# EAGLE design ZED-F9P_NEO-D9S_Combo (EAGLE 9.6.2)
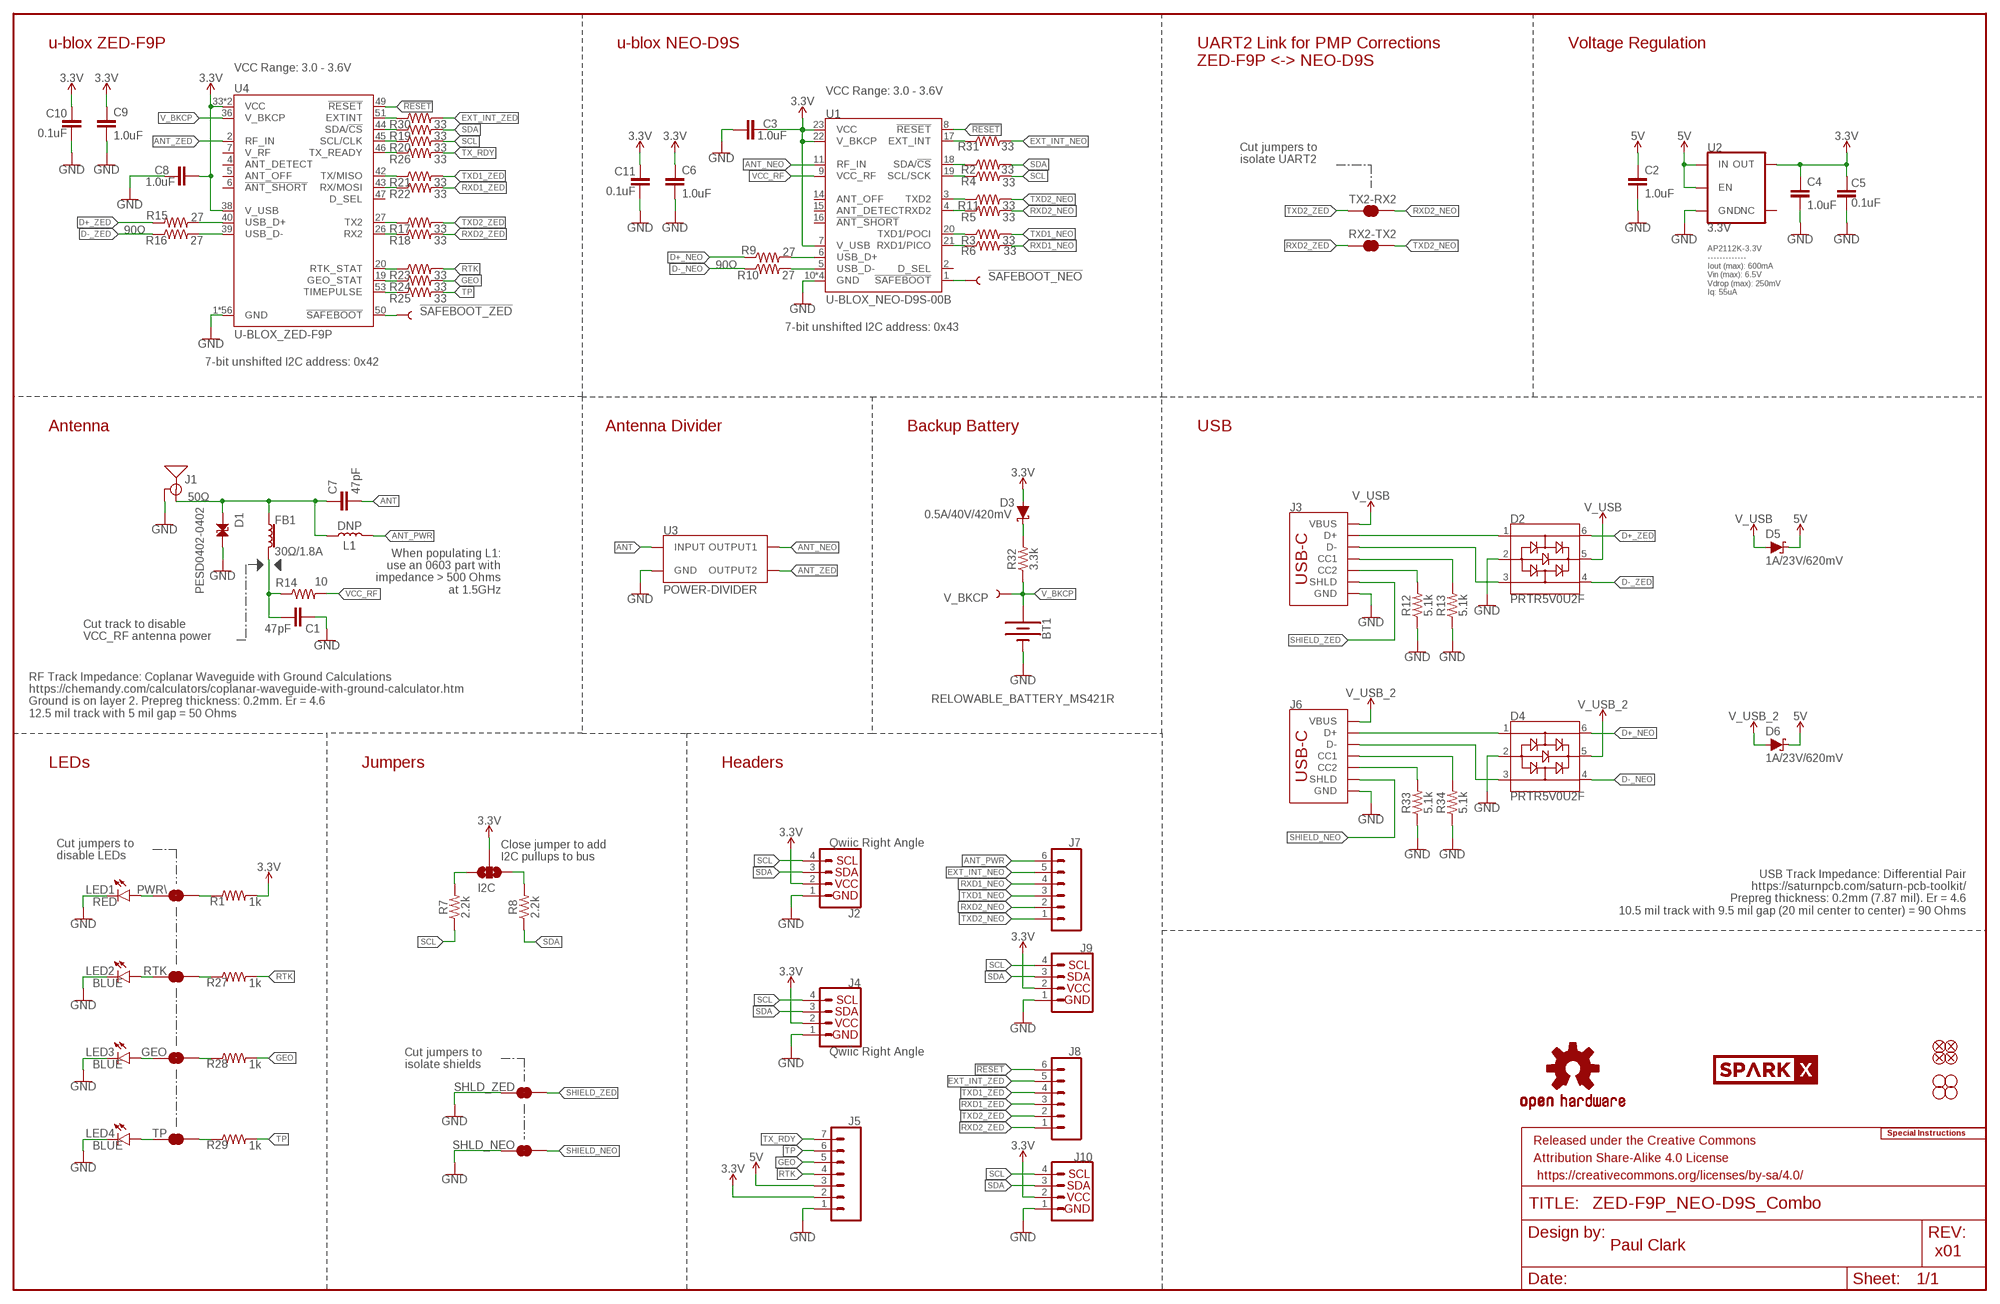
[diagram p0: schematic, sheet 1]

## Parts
!SAFEBOOT_NEO!  TEST-POINTPOGO_PTH  [1X01_NO_SILK]
!SAFEBOOT_ZED!  TEST-POINTPOGO_PTH  [1X01_NO_SILK]
BT1  RELOWABLE_BATTERY_MS421R  [MS421R_IV03E]
C1  47pF  47PF-0603-50V-5%  [0603]
C2  1.0uF  1.0UF-0603-16V-10%  [0603]
C3  1.0uF  1.0UF-0603-16V-10%  [0603]
C4  1.0uF  1.0UF-0603-16V-10%  [0603]
C5  0.1uF  0.1UF-0603-25V-(+80/-20%)  [0603]
C6  1.0uF  1.0UF-0603-16V-10%  [0603]
C7  47pF  47PF-0603-50V-5%  [0603]
C8  1.0uF  1.0UF-0603-16V-10%  [0603]
C9  1.0uF  1.0UF-0603-16V-10%  [0603]
C10  0.1uF  0.1UF-0603-25V-(+80/-20%)  [0603]
C11  0.1uF  0.1UF-0603-25V-(+80/-20%)  [0603]
D1  PESD0402-0402  [0402]
D2  PRTR5V0U2F  [SOT886]
D3  0.5A/40V/420mV  DIODE-SCHOTTKY-PMEG4005EJ  [SOD-323]
D4  PRTR5V0U2F  [SOT886]
D5  1A/23V/620mV  DIODE-SCHOTTKY-BAT20J  [SOD-323]
D6  1A/23V/620mV  DIODE-SCHOTTKY-BAT20J  [SOD-323]
FB1  30Ω/1.8A  FERRITE_BEAD-0603  [0603]
FRAME2  FRAME-LEDGER  [CREATIVE_COMMONS]
GEO  JUMPER-SMT_2_NC_TRACE_SILK  [SMT-JUMPER_2_NC_TRACE_SILK]
I2C  JUMPER-SMT_3_NO_SILK  [SMT-JUMPER_3_NO_SILK]
J1  ANTENNA-SMA-GROUNDEDEDGE_SMA  [SMA-EDGE]
J2  Qwiic Right Angle  I2C_STANDARDQWIIC  [JST04_1MM_RA]
J3  USB Female Type C Connector  USB_C_4-LAYER_PADS  [USB-C-16P_4LAYER-PADS]
J4  Qwiic Right Angle  I2C_STANDARDQWIIC  [JST04_1MM_RA]
J5  CONN_07NO_SILK  [1X07_NO_SILK]
J6  USB Female Type C Connector  USB_C_4-LAYER_PADS  [USB-C-16P_4LAYER-PADS]
J7  CONN_06NO_SILK_FEMALE_PTH  [1X06_NO_SILK]
J8  CONN_06NO_SILK_FEMALE_PTH  [1X06_NO_SILK]
J9  I2C_STANDARD_NO_SILK  [1X04_NO_SILK]
J10  I2C_STANDARD_NO_SILK  [1X04_NO_SILK]
JP21  FIDUCIALUFIDUCIAL  [MICRO-FIDUCIAL]
JP31  STAND-OFF  [STAND-OFF]
JP41  STAND-OFF  [STAND-OFF]
JP61  FIDUCIALUFIDUCIAL  [MICRO-FIDUCIAL]
JP71  FIDUCIALUFIDUCIAL  [MICRO-FIDUCIAL]
JP81  FIDUCIALUFIDUCIAL  [MICRO-FIDUCIAL]
JP91  STAND-OFF  [STAND-OFF]
JP101  STAND-OFF  [STAND-OFF]
L1  DNP  DNP-0603_NO-CREAM  [0603_NO-CREAM]
LED1  RED  LED-RED0603  [LED-0603]
LED2  BLUE  LED-BLUE0603  [LED-0603]
LED3  BLUE  LED-BLUE0603  [LED-0603]
LED4  BLUE  LED-BLUE0603  [LED-0603]
LOGO4  OSHW-LOGOS  [OSHW-LOGO-S]
LOGO5  SPECIAL_INSTRUCTIONS-ORDERING  [ORDERING_INSTRUCTIONS]
PWR\  JUMPER-SMT_2_NC_TRACE_SILK  [SMT-JUMPER_2_NC_TRACE_SILK]
R1  1k  1KOHM-0603-1/10W-1%  [0603]
R2  33  33OHM-0603-1/10W-1%  [0603]
R3  33  33OHM-0603-1/10W-1%  [0603]
R4  33  33OHM-0603-1/10W-1%  [0603]
R5  33  33OHM-0603-1/10W-1%  [0603]
R6  33  33OHM-0603-1/10W-1%  [0603]
R7  2.2k  2.2KOHM-0603-1/10W-1%  [0603]
R8  2.2k  2.2KOHM-0603-1/10W-1%  [0603]
R9  27  27OHM-0603-1/10W-1%  [0603]
R10  27  27OHM-0603-1/10W-1%  [0603]
R11  33  33OHM-0603-1/10W-1%  [0603]
R12  5.1k  5.1KOHM5.1KOHM-0603-1/10W-1%  [0603]
R13  5.1k  5.1KOHM5.1KOHM-0603-1/10W-1%  [0603]
R14  10  10OHM-0603-1/10W-1%  [0603]
R15  27  27OHM-0603-1/10W-1%  [0603]
R16  27  27OHM-0603-1/10W-1%  [0603]
R17  33  33OHM-0603-1/10W-1%  [0603]
R18  33  33OHM-0603-1/10W-1%  [0603]
R19  33  33OHM-0603-1/10W-1%  [0603]
R20  33  33OHM-0603-1/10W-1%  [0603]
R21  33  33OHM-0603-1/10W-1%  [0603]
R22  33  33OHM-0603-1/10W-1%  [0603]
R23  33  33OHM-0603-1/10W-1%  [0603]
R24  33  33OHM-0603-1/10W-1%  [0603]
R25  33  33OHM-0603-1/10W-1%  [0603]
R26  33  33OHM-0603-1/10W-1%  [0603]
R27  1k  1KOHM-0603-1/10W-1%  [0603]
R28  1k  1KOHM-0603-1/10W-1%  [0603]
R29  1k  1KOHM-0603-1/10W-1%  [0603]
R30  33  33OHM-0603-1/10W-1%  [0603]
R31  33  33OHM-0603-1/10W-1%  [0603]
R32  3.3k  3.3KOHM-0603-1/10W-1%  [0603]
R33  5.1k  5.1KOHM5.1KOHM-0603-1/10W-1%  [0603]
R34  5.1k  5.1KOHM5.1KOHM-0603-1/10W-1%  [0603]
RTK  JUMPER-SMT_2_NC_TRACE_SILK  [SMT-JUMPER_2_NC_TRACE_SILK]
RX2-TX2  JUMPER-SMT_2_NC_TRACE_SILK  [SMT-JUMPER_2_NC_TRACE_SILK]
SHLD_NEO  JUMPER-SMT_2_NC_TRACE_SILK  [SMT-JUMPER_2_NC_TRACE_SILK]
SHLD_ZED  JUMPER-SMT_2_NC_TRACE_SILK  [SMT-JUMPER_2_NC_TRACE_SILK]
TP  JUMPER-SMT_2_NC_TRACE_SILK  [SMT-JUMPER_2_NC_TRACE_SILK]
TX2-RX2  JUMPER-SMT_2_NC_TRACE_SILK  [SMT-JUMPER_2_NC_TRACE_SILK]
U1  U-BLOX_NEO-D9S-00B  [NEO-M9N/M8T/M8U/D9S]
U2  3.3V  V_REG_AP2112K-3.3V  [SOT23-5]
U3  POWER-DIVIDER  [PD0922J5050S2HF_ANA]
U4  U-BLOX_ZED-F9P  [ZED-F9P]
U$77  SPARKX-LOGO4  [SPARKX-MEDIUM]
U$78  SPARKX-LOGO4  [SPARKX-MEDIUM]
V_BKCP  TEST-POINT3X5  [PAD.03X.05]

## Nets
3.3V [3.3V]: C3.1 C4.1 C5.2 C6.1 C8.2 C9.1 C10.2 C11.2 D3.A I2C.2 J2.2 J4.2 J5.2 J9.2 J10.2 R1.2 U1.7(V_USB) U1.22(V_BKCP) U1.23(VCC) U2.5(OUT) U4.33(VCC) U4.34(VCC) U4.38(V_USB)
5V: C2.1 D5.C D6.C J5.3 U2.1(IN) U2.3(EN)
!RESET!: J8.6 U1.8(!RESET!) U4.49(!RESET!)
!SAFEBOOT_NEO!: !SAFEBOOT_NEO!.1 U1.1(!SAFEBOOT!)
!SAFEBOOT_ZED!: !SAFEBOOT_ZED!.1 U4.50(!SAFEBOOT!)
ANT: C7.2 U3.2(INPUT)
ANT_NEO: U1.11(RF_IN) U3.4(OUTPUT1)
ANT_PWR: J7.6 L1.2
ANT_VCC: C1.1 FB1.2 R14.1
ANT_ZED: U3.6(OUTPUT2) U4.2(RF_IN)
D+_NEO: D4.6 R9.1
D+_ZED: D2.6 R15.1
D-_NEO: D4.4 R10.1
D-_ZED: D2.4 R16.1
EXT_INT_NEO: J7.5 R31.2
EXT_INT_ZED: J8.5 R30.2
GEO: J5.5 R24.2 R28.2
GND: BT1.- C1.2 C2.2 C3.2 C4.2 C5.1 C6.2 C8.1 C9.2 C10.1 C11.1 D1.2 D2.2 D4.2 J1.GND@0(GND) J1.GND@1(GND) J1.GND@2(GND) J1.GND@3(GND) J2.1 J3.GND J3.GND2(GND) J4.1 J5.1 J6.GND J6.GND2(GND) J9.1 J10.1 LED1.C LED2.C LED3.C LED4.C R12.1 R13.1 R33.1 R34.1 SHLD_NEO.1 SHLD_ZED.1 U1.10(GND) U1.12(GND) U1.13(GND) U1.24(GND) U2.2(GND) U3.1(GND) U3.3(GND) U3.5(GND) U4.1(GND) U4.3(GND) U4.12(GND) U4.14(GND) U4.32(GND) U4.37(GND) U4.41(GND) U4.48(GND) U4.55(GND) U4.56(GND) U4.57(GND) U4.58(GND) U4.59(GND) U4.60(GND) U4.61(GND) U4.62(GND) U4.63(GND) U4.64(GND) U4.65(GND) U4.66(GND) U4.67(GND) U4.68(GND) U4.69(GND) U4.70(GND) U4.71(GND) U4.72(GND) U4.73(GND) U4.74(GND) U4.75(GND) U4.76(GND) U4.77(GND) U4.78(GND) U4.79(GND) U4.80(GND) U4.81(GND) U4.82(GND) U4.83(GND) U4.84(GND) U4.85(GND) U4.86(GND) U4.87(GND) U4.88(GND) U4.89(GND) U4.90(GND) U4.91(GND) U4.92(GND) U4.93(GND) U4.94(GND) U4.95(GND) U4.96(GND) U4.97(GND) U4.98(GND) U4.99(GND) U4.100(GND) U4.101(GND) U4.102(GND)
N$1: PWR\.2 R1.1
N$2: R3.1 U1.20(TXD1/POCI)
N$3: R2.1 U1.18(SDA/!CS!)
N$4: R4.1 U1.19(SCL/SCK)
N$5: I2C.1 R8.2
N$6: R6.1 U1.21(RXD1/PICO)
N$7: J3.B5(CC2) R12.2
N$8: I2C.3 R7.2
N$9: J3.A5(CC1) R13.2
N$10: LED1.A PWR\.1
N$11: R9.2 U1.6(USB_D+)
N$12: R10.2 U1.5(USB_D-)
N$13: D3.C R32.2
N$14: R11.1 U1.3(TXD2)
N$15: R5.1 U1.4(RXD2)
N$16: R15.2 U4.40(USB_D+)
N$17: R16.2 U4.39(USB_D-)
N$18: R19.1 U4.44(SDA/!CS!)
N$19: R20.1 U4.45(SCL/CLK)
N$20: R21.1 U4.42(TX/MISO)
N$21: R22.1 U4.43(RX/MOSI)
N$22: R26.1 U4.46(TX_READY)
N$23: LED2.A RTK.1
N$24: R17.1 U4.27(TX2)
N$25: R18.1 U4.26(RX2)
N$26: GEO.1 LED3.A
N$27: LED4.A TP.1
N$28: R27.1 RTK.2
N$29: GEO.2 R28.1
N$30: R29.1 TP.2
N$31: R30.1 U4.51(EXTINT)
N$32: R31.1 U1.17(EXT_INT)
N$33: J6.B5(CC2) R33.2
N$34: J6.A5(CC1) R34.2
N$35: R23.1 U4.20(RTK_STAT)
N$36: R24.1 U4.19(GEO_STAT)
N$37: R25.1 U4.53(TIMEPULSE)
RTK: J5.4 R23.2 R27.2
RXD1_NEO: J7.4 R6.2
RXD1_ZED: J8.3 R22.2
RXD2_NEO: J7.2 R5.2 TX2-RX2.2
RXD2_ZED: J8.1 R18.2 RX2-TX2.1
SCL: J2.4 J4.4 J9.4 J10.4 R4.2 R7.1 R20.2
SDA: J2.3 J4.3 J9.3 J10.3 R2.2 R8.1 R19.2
SHIELD_NEO: J6.SHLD1(SHLD) J6.SHLD2(SHLD) J6.SHLD3(SHLD) J6.SHLD4(SHLD) SHLD_NEO.2
SHIELD_ZED: J3.SHLD1(SHLD) J3.SHLD2(SHLD) J3.SHLD3(SHLD) J3.SHLD4(SHLD) SHLD_ZED.2
SMA: C7.1 D1.1 FB1.1 J1.SIG(SIGNAL) L1.1
TP: J5.6 R25.2 R29.2
TX_RDY: J5.7 R26.2
TXD1_NEO: J7.3 R3.2
TXD1_ZED: J8.4 R21.2
TXD2_NEO: J7.1 R11.2 RX2-TX2.2
TXD2_ZED: J8.2 R17.2 TX2-RX2.1
USB_D+: D2.1 J3.A6(D+) J3.B6(D+)
USB_D+1: D4.1 J6.A6(D+) J6.B6(D+)
USB_D-: D2.3 J3.A7(D-) J3.B7(D-)
USB_D-1: D4.3 J6.A7(D-) J6.B7(D-)
V_BKCP: BT1.+ R32.1 U4.36(V_BKCP) V_BKCP.1
V_USB: D2.5 D5.A J3.VBUS1(VBUS) J3.VBUS2(VBUS)
V_USB_2: D4.5 D6.A J6.VBUS1(VBUS) J6.VBUS2(VBUS)
VCC_RF: R14.2 U1.9(VCC_RF)
Unconnected: U1.2(D_SEL) U1.14(ANT_OFF) U1.15(ANT_DETECT) U1.16(!ANT_SHORT!) U2.4(NC) U4.4(ANT_DETECT) U4.5(ANT_OFF) U4.6(!ANT_SHORT!) U4.7(V_RF) U4.47(D_SEL)

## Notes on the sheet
- UART2 Link for PMP Corrections
  ZED-F9P <-> NEO-D9S
- u-blox ZED-F9P | u-blox NEO-D9S | Voltage Regulation
- VCC Range: 3.0 - 3.6V
- VCC Range: 3.0 - 3.6V
- Cut jumpers to
  isolate UART2
- 90Ω
- AP2112K-3.3V
  -------------
  Iout (max): 600mA 
  Vin (max): 6.5V
  Vdrop (max): 250mV
  Iq: 55uA
- 90Ω
- 7-bit unshifted I2C address: 0x43
- 7-bit unshifted I2C address: 0x42
- Antenna | Antenna Divider | Backup Battery | USB
- 50Ω
- When populating L1:
  use an 0603 part with
  impedance > 500 Ohms
  at 1.5GHz
- Cut track to disable
  VCC_RF antenna power
- RF Track Impedance: Coplanar Waveguide with Ground Calculations
  https://chemandy.com/calculators/coplanar-waveguide-with-ground-calculator.htm
  Ground is on layer 2. Prepreg thickness: 0.2mm. Er = 4.6
  12.5 mil track with 5 mil gap = 50 Ohms
- LEDs | Jumpers | Headers
- Cut jumpers to 
  disable LEDs
- Close jumper to add
  I2C pullups to bus
- USB Track Impedance: Differential Pair
  https://saturnpcb.com/saturn-pcb-toolkit/
  Prepreg thickness: 0.2mm (7.87 mil). Er = 4.6
  10.5 mil track with 9.5 mil gap (20 mil center to center) = 90 Ohms
- Cut jumpers to 
  isolate shields
- Paul Clark
- x01

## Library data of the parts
!SAFEBOOT_NEO! !SAFEBOOT_ZED! V_BKCP = SparkFun-Connectors:TEST-POINT: SparkFun Test Points
BT1 = SparkFun-Batteries:RELOWABLE_BATTERY: SEIKO Reflowable Lithium Batteries; PROD_ID: BAT-16685
C1 C7 = SparkFun-Capacitors:47PF: 47pF ceramic capacitors; PROD_ID: CAP-08913
C2-C4 C6 C8 C9 = SparkFun-Capacitors:1.0UF: 1µF ceramic capacitors; PROD_ID: CAP-00868
C5 C10 C11 = SparkFun-Capacitors:0.1UF: 0.1µF ceramic capacitors; PROD_ID: CAP-00810
D1 = SparkFun-DiscreteSemi:PESD0402: ESD protection diode; DIGIKEY_PART: PESD0402-140CT-ND; MOUSE_PART: 650-PESD0402-140; PROD_ID: DIO-15359
D2 D4 = SparkFun-IC-Power:PRTR5V0U2: A small ESD protection device. Most commonly used on USB D+/D- signals to protect large, expensive, or especially sensitive USB enabled devices.; PROD_ID: DIO-14084
D3 = SparkFun-DiscreteSemi:DIODE-SCHOTTKY: Schottky diode; PROD_ID: DIO-10955
D5 D6 = SparkFun-DiscreteSemi:DIODE-SCHOTTKY: Schottky diode; PROD_ID: DIO-11623
FB1 = SparkFun-Coils:FERRITE_BEAD: Ferrite Bead (blocks, cores, rings, chokes, etc.); PROD_ID: NDUC-13805
FRAME2 = SparkFun-Aesthetics:FRAME-LEDGER: Schematic Frame - Ledger
GEO PWR\ RTK RX2-TX2 SHLD_NEO SHLD_ZED TP TX2-RX2 = SparkFun-Jumpers:JUMPER-SMT_2_NC_TRACE: Normally closed trace jumper
I2C = SparkFun-Jumpers:JUMPER-SMT_3_NO: Normally open jumper This jumper has three pads in close proximity to each other. Apply solder to close the connection(s).
J1 = SparkFun-RF:ANTENNA-SMA-GROUNDED: SMA Antenna Connector w/ Ground; PROD_ID: CONN-08289
J2 J4 = SparkFun-Connectors:I2C_STANDARD: SparkFun I2C Standard Pinout Header SparkFun has standardized on a pinout for all I2C based sensor breakouts. This pinout allows I2C boards to be plugged directly into the headers on Arduino Uno compatible boards, and to be daisy chained easily. Example SparkFun Products: SparkFun Atmospheric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; PROD_ID: CONN-13694
J3 J6 = SparkFun-Connectors:USB_C: USB Type C 16Pin Connector Super Speed pins not available on the 16-pin purely SMD connector so this part is best for USB 2.0 implementations. D1 and D2 are tied together enabling D+/- no matter which way the cable is plugged into the connector. The two channel configuration pins (CC1/2) are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; PROD_ID: CONN-14122
J5 = SparkFun-Connectors:CONN_07: Multi connection point. Often used as Generic Header-pin footprint for 0.1 inch spaced/style header connections On any of the 0.1 inch spaced packages, you can populate with these: Break Away Headers - Straight (PRT-00116) Break Away Male Headers - Right Angle (PRT-00553) Female Headers (PRT-00115)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
J7 J8 = SparkFun-Connectors:CONN_06: Multi connection point. Often used as Generic Header-pin footprint for 0.1 inch spaced/style header connections On any of the 0.1 inch spaced packages, you can populate with these: Break Away Headers - Straight (PRT-00116) Break Away Male Headers - Right Angle (PRT-00553) Female Headers (PRT-00115)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; PROD_ID: CONN-08437
J9 J10 = SparkFun-Connectors:I2C_STANDARD: SparkFun I2C Standard Pinout Header SparkFun has standardized on a pinout for all I2C based sensor breakouts. This pinout allows I2C boards to be plugged directly into the headers on Arduino Uno compatible boards, and to be daisy chained easily. Example SparkFun Products: SparkFun Atmospheric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
JP21 JP61 JP71 JP81 = SparkFun:FIDUCIAL: Fiducial Alignment Points
JP31 JP41 JP91 JP101 = SparkFun:STAND-OFF: Stand Off
L1 = SparkFun-Coils:DNP
LED1 = SparkFun-LED:LED-RED: Red SMD LED; PROD_ID: DIO-00819
LED2-LED4 = SparkFun-LED:LED-BLUE: Blue SMD LED; PROD_ID: DIO-08575
LOGO4 = SparkFun-Aesthetics:OSHW-LOGO: Open-Source Hardware (OSHW) Logo
LOGO5 = SparkFun-Aesthetics:SPECIAL_INSTRUCTIONS: Special Ordering/Production Instructions Alert
R1 R27-R29 = SparkFun-Resistors:1KOHM: 1kΩ resistor; PROD_ID: RES-07856
R2-R6 R11 R17-R26 R30 R31 = SparkFun-Resistors:33OHM: 33Ω resistor; PROD_ID: RES-08270
R7 R8 = SparkFun-Resistors:2.2KOHM: 2.2kΩ resistor; PROD_ID: RES-08272
R9 R10 R15 R16 = SparkFun-Resistors:27OHM: 27Ω resistor; PROD_ID: RES-09334
R12 R13 R33 R34 = SparkFun-Resistors:5.1KOHM; PROD_ID: RES-12083
R14 = SparkFun-Resistors:10OHM: 10Ω resistor; PROD_ID: RES-12581
R32 = SparkFun-Resistors:3.3KOHM: 3.3kΩ resistor; PROD_ID: RES-07851
U1 = SparkFun-GPS:U-BLOX_NEO-D9S: u-blox NEO-D9S The NEO-D9S can receive the data stream of a GNSS correction service, broadcast via satellite L band and compliant to the specification the product is designed for. Integrated with a high precision GNSS receiver, such as from the u-blox F9 platform, it enables the positioning system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; PROD_ID: IC-16579
U2 = SparkFun-IC-Power:V_REG_AP2112: AP2112 - 600mA CMOS LDO Regulator w/ Enable The AP2112 is CMOS process low dropout linear regulator with enable function, the regulator delivers a guaranteed 600mA (min.) continuous load current. Features Output Voltage Accuracy: ±1.5% Output Current: 600mA (Min.) Foldback Short Current Protection: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; PROD_ID: VREG-12457
U3 = SparkFun-GPS:POWER-DIVIDER: The PD0922J5050S2HF is a low profile, sub-miniature Wilkinson power divider in an easy to use surface mount package. The PD0922J5050S2HF is matched to 50 Ω and has a height profile of 0.5 mm which is ideal for high level integrations in the following markets: DVB-S, DVB-H (USA), GSM, DCS, PCS,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; MANUFACTURER_PART_NUMBER: PD0922J5050S2HF; PROD_ID: IC-16658
U4 = SparkFun-GPS:U-BLOX_ZED-F9P; PROD_ID: IC-14209
U$77 U$78 = SparkX:SPARKX-LOGO

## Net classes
1 vcc: width 0.152 mm
2 3.3V: width 0.508 mm
4 DiffPair: width 0.152 mm, clearance 0.178 mm

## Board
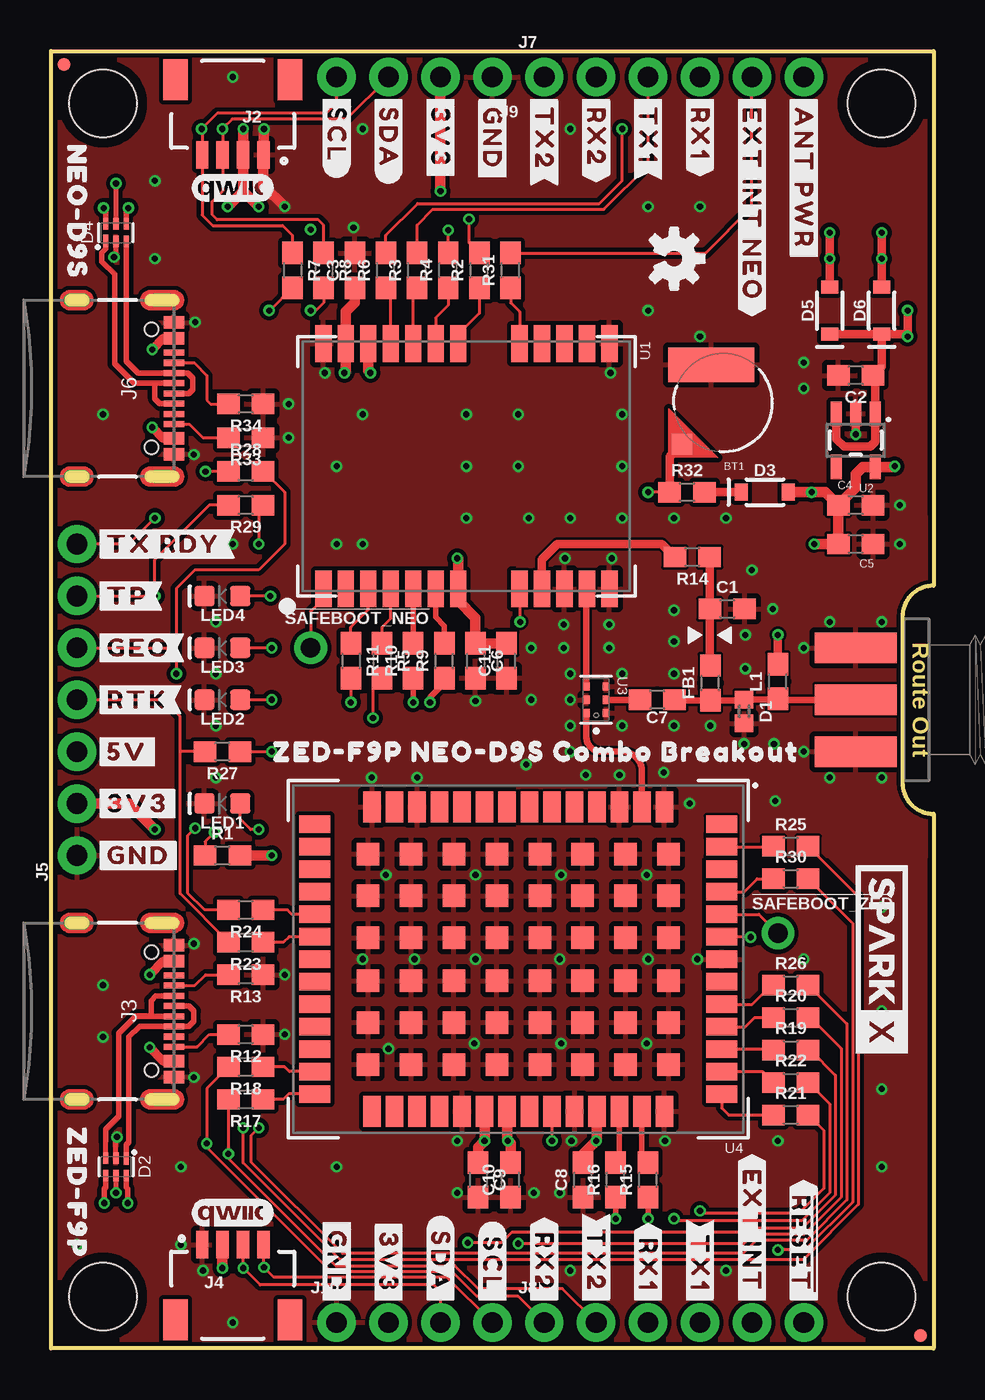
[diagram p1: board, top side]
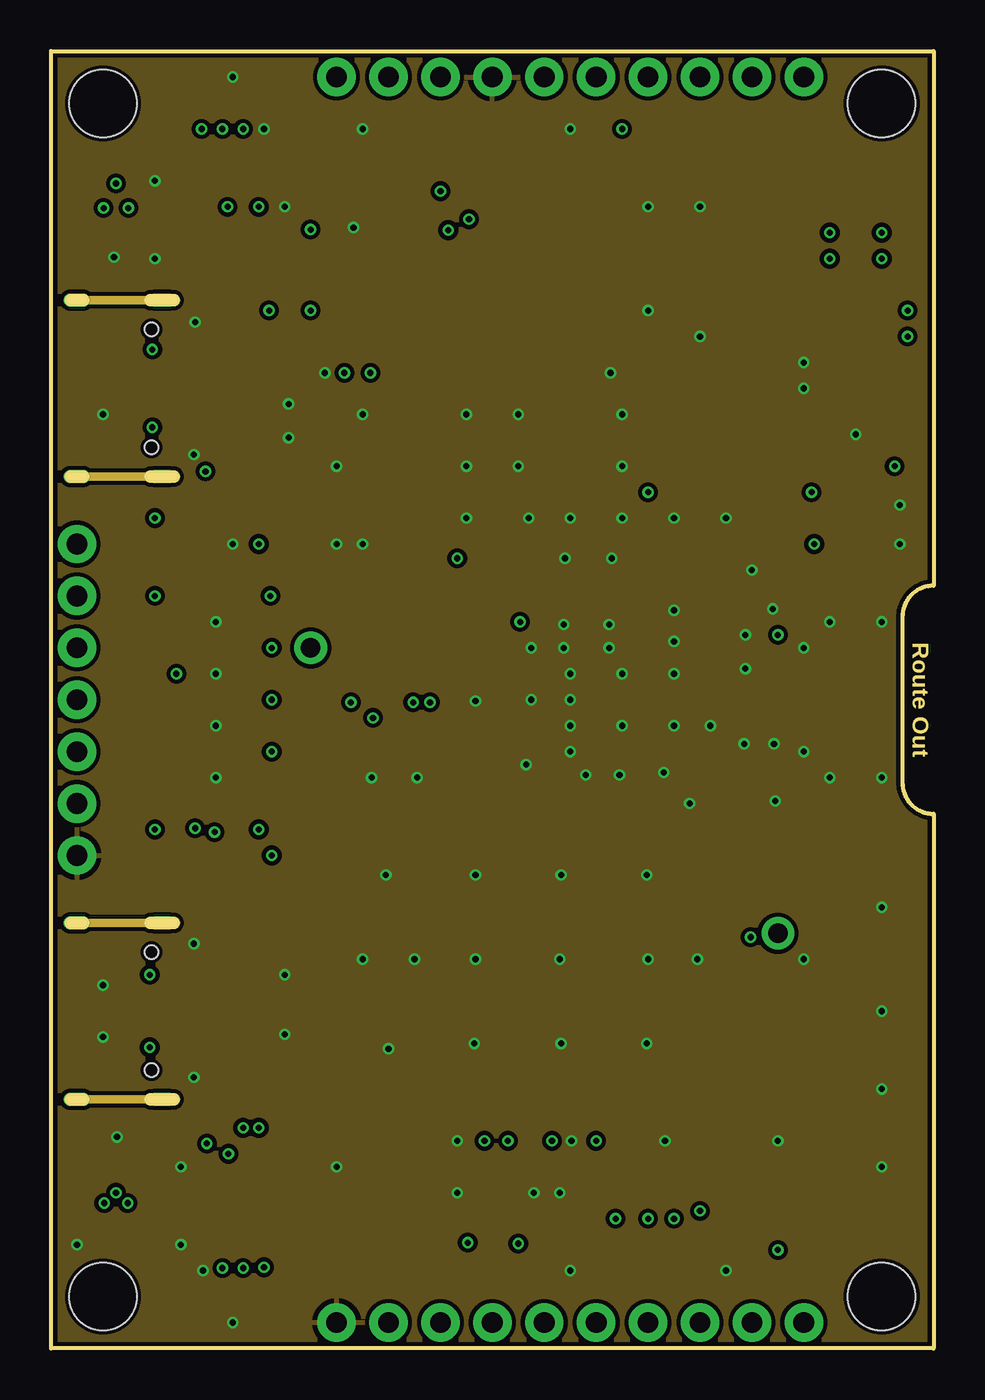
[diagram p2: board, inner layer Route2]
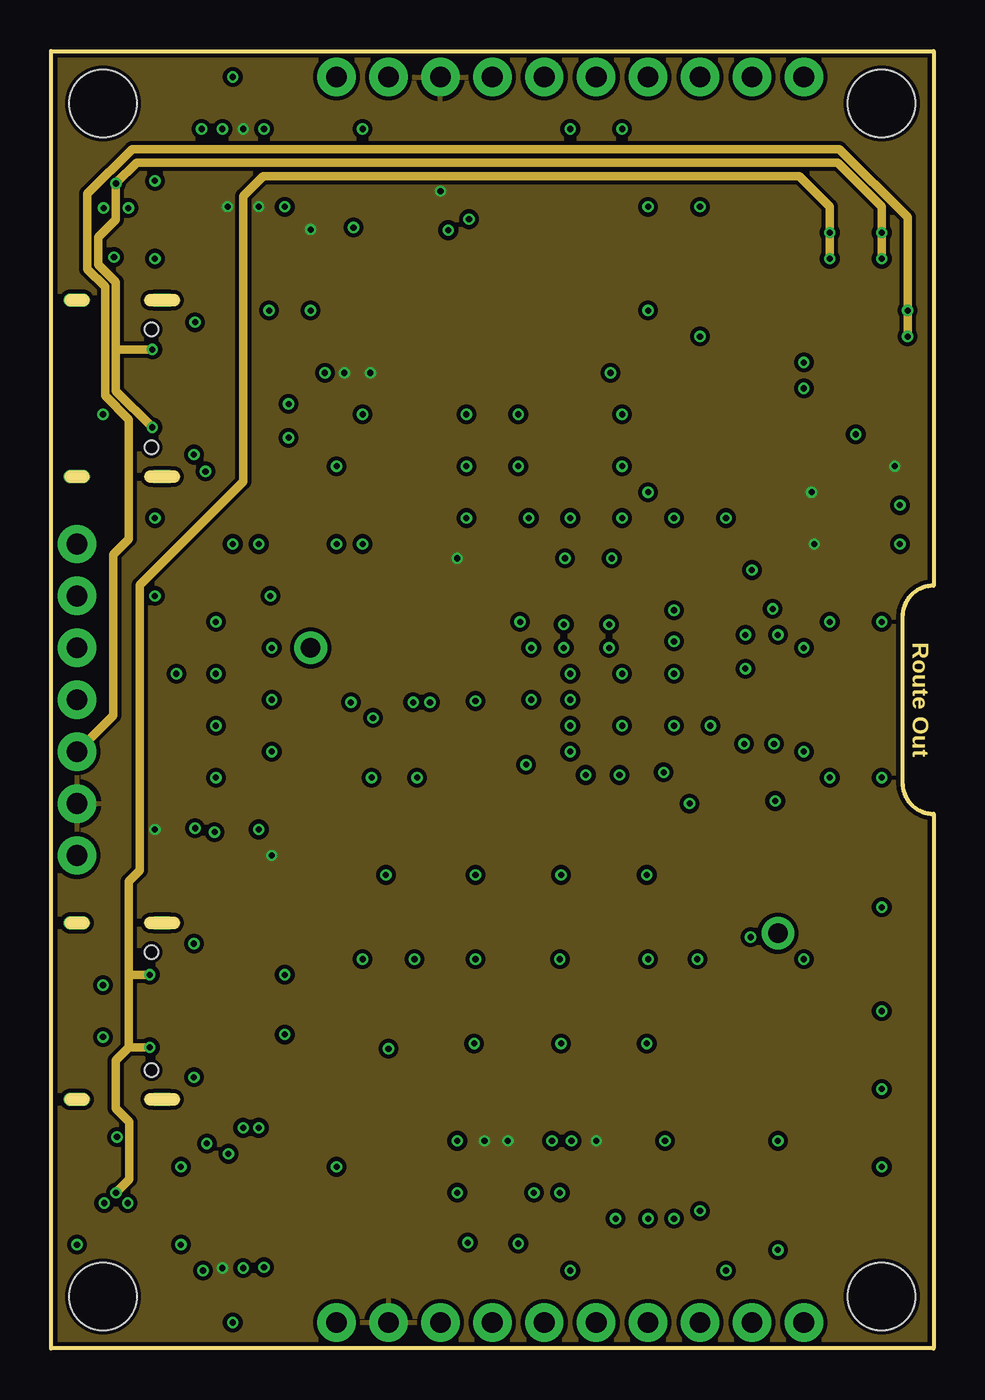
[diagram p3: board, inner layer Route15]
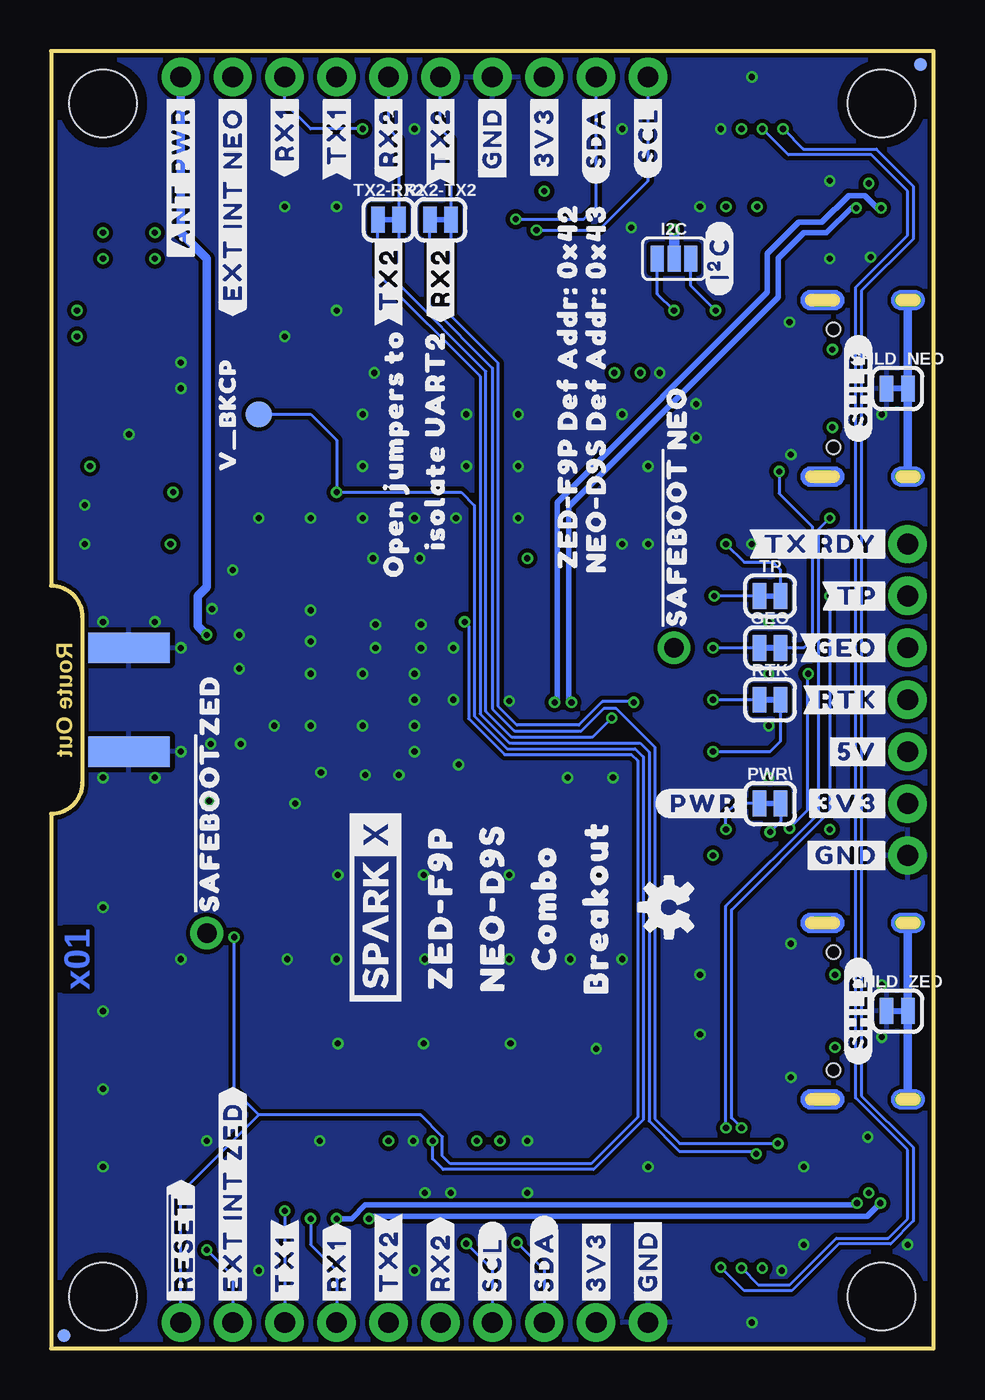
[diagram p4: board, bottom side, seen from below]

Size 43.18 x 63.5 mm. Coordinates in mm from the lower left corner, seen from the top.
Outline: 0,0 0,63.5 43.18,63.5 43.18,37.34 arc90 41.66,35.81 41.66,27.69 arc90 43.18,26.16 43.18,0 0,0
Copper layers (1*2*15*16): Top 0.035559375mm / dielectric 0.47751875mm / Route2 0.035559375mm / dielectric 0.47751875mm / Route15 0.035559375mm / dielectric 0.47751875mm / Bottom 0.035559375mm
Design rules "SparkFun-4-Layer-Minimum-JLCPCB": minimum track width 5mil, minimum drill 0.2mm, track to track 5mil, track to pad 5mil, pad to pad 5mil, via to via 5mil, smd to smd 5mil, copper to edge 7mil, drill to drill 7mil, minimum pad ring 5mil, minimum via ring 5mil, stop-mask expansion 2.5mil, vias tented up to drill 25mil, thermal gap 10mil
tRestrict: 4 lines

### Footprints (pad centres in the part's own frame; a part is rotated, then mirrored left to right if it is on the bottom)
1X01_NO_SILK = drill 0.95 pad 1.6: 1 0,0
MS421R_IV03E = smd 1 x 1: + 2.022,2.032 | smd 4.2 x 1.7: - 0.6,-1.85
0603 = smd 1.1 x 1: 1 -0.85,0; 2 0.85,0
0402 = smd 0.85 x 0.9: 1 -0.58,0; 2 0.58,0
SOT886 = smd 0.61 x 0.25: 1 -0.405,0.5 | smd 0.56 x 0.25: 2 -0.43,0; 3 -0.43,-0.5; 4 0.43,-0.5; 5 0.43,0; 6 0.43,0.5
SOD-323 = smd 0.63 x 0.83: A 1.15,0; C -1.15,0
SMT-JUMPER_2_NC_TRACE_SILK = smd 0.66 x 1.27: 1 -0.521,0; 2 0.521,0
SMT-JUMPER_3_NO_SILK = smd 0.635 x 1.27: 1 -0.813,0; 2 0,0; 3 0.813,0
SMA-EDGE = smd 1.5 x 4: GND@0 -2.54,0; GND@1 2.54,0; SIG 0,0 | smd 1.5 x 4 bottom: GND@2 -2.54,0; GND@3 2.54,0
JST04_1MM_RA = smd 0.6 x 1.35: 1 -1.5,0; 2 -0.5,0; 3 0.5,0; 4 1.5,0 | smd 1.2 x 2: NC1 2.8,-3.675; NC2 -2.8,-3.675
USB-C-16P_4LAYER-PADS = smd 0.3 x 1: A5 -1.25,-0.34; A6 -0.25,-0.34; A7 0.25,-0.34; A8 1.25,-0.34; B5 1.75,-0.34; B6 0.75,-0.34; B7 -0.75,-0.34; B8 -1.75,-0.34 | smd 0.6 x 1: GND -3.225,-0.34; GND2 3.225,-0.34; VBUS1 -2.45,-0.34; VBUS2 2.45,-0.34 | drill 0.4 pad 0.6 long: SHLD1 -4.318,-0.915; SHLD2 4.318,-0.915; SHLD3 -4.318,-5.095; SHLD4 4.318,-5.095 | hole 0.65: -2.89,-1.445; 2.89,-1.445
1X07_NO_SILK = drill 1.016 pad 1.88: 1 0,0; 2 2.54,0; 3 5.08,0; 4 7.62,0; 5 10.16,0; 6 12.7,0; 7 15.24,0
1X06_NO_SILK = drill 1.016 pad 1.88: 1 0,0; 2 2.54,0; 3 5.08,0; 4 7.62,0; 5 10.16,0; 6 12.7,0
1X04_NO_SILK = drill 1.016 pad 1.88: 1 0,0; 2 2.54,0; 3 5.08,0; 4 7.62,0
MICRO-FIDUCIAL = smd 0.635 x 0.635: 1 0,0
STAND-OFF = hole 3.302: 0,0
0603_NO-CREAM = smd 1.1 x 1: 1 -0.85,0; 2 0.85,0
LED-0603 = smd 1 x 1: A -0.877,0; C 0.877,0
NEO-M9N/M8T/M8U/D9S = smd 1.8 x 0.8: 1 6,-7; 2 6,-5.9; 3 6,-4.8; 4 6,-3.7; 5 6,-2.6; 6 6,-1.5; 7 6,-0.4; 8 6,2.6; 9 6,3.7; 10 6,4.8; 11 6,5.9; 12 6,7; 13 -6,7; 14 -6,5.9; 15 -6,4.8; 16 -6,3.7; 17 -6,2.6; 18 -6,-0.4; 19 -6,-1.5; 20 -6,-2.6; 21 -6,-3.7; 22 -6,-4.8; 23 -6,-5.9; 24 -6,-7
SOT23-5 = smd 0.55 x 1.2: 1 -0.95,-1.3; 2 0,-1.3; 3 0.95,-1.3; 4 0.95,1.3; 5 -0.95,1.3
PD0922J5050S2HF_ANA = smd 0.41 x 0.33: 1 0.65,0.483; 2 0,0.483; 3 -0.65,0.483; 4 -0.65,-0.483; 5 0,-0.483; 6 0.65,-0.483
ZED-F9P = smd 0.85 x 1.52: 1 -7.15,-7.45; 2 -6.05,-7.45; 3 -4.95,-7.45; 4 -3.85,-7.45; 5 -2.75,-7.45; 6 -1.65,-7.45; 7 -0.55,-7.45; 8 0.55,-7.45; 9 1.65,-7.45; 10 2.75,-7.45; 11 3.85,-7.45; 12 4.95,-7.45; 13 6.05,-7.45; 14 7.15,-7.45; 28 7.15,7.45; 29 6.05,7.45; 30 4.95,7.45; 31 3.85,7.45; 32 2.75,7.45; 33 1.65,7.45; 34 0.55,7.45; 35 -0.55,7.45; 36 -1.65,7.45; 37 -2.75,7.45; 38 -3.85,7.45; 39 -4.95,7.45; 40 -6.05,7.45; 41 -7.15,7.45 | smd 1.52 x 0.85: 15 9.95,-6.6; 16 9.95,-5.5; 17 9.95,-4.4; 18 9.95,-3.3; 19 9.95,-2.2; 20 9.95,-1.1; 21 9.95,0; 22 9.95,1.1; 23 9.95,2.2; 24 9.95,3.3; 25 9.95,4.4; 26 9.95,5.5; 27 9.95,6.6; 42 -9.95,6.6; 43 -9.95,5.5; 44 -9.95,4.4; 45 -9.95,3.3; 46 -9.95,2.2; 47 -9.95,1.1; 48 -9.95,0; 49 -9.95,-1.1; 50 -9.95,-2.2; 51 -9.95,-3.3; 52 -9.95,-4.4; 53 -9.95,-5.5; 54 -9.95,-6.6 | smd 1.1 x 1.1: 55 -1.05,-1.05; 56 -3.15,-1.05; 57 -5.25,-1.05; 58 -7.35,-1.05; 59 -1.05,-3.1; 60 -3.15,-3.1; 61 -5.25,-3.1; 62 -7.35,-3.1; 63 -1.05,-5.15; 64 -3.15,-5.15; 65 -5.25,-5.15; 66 -7.35,-5.15; 67 -1.05,5.15; 68 -3.15,5.15; 69 -5.25,5.15; 70 -7.35,5.15; 71 -1.05,3.1; 72 -3.15,3.1; 73 -5.25,3.1; 74 -7.35,3.1; 75 -1.05,1.05; 76 -3.15,1.05; 77 -5.25,1.05; 78 -7.35,1.05; 79 1.05,1.05; 80 3.15,1.05; 81 5.25,1.05; 82 7.35,1.05; 83 1.05,3.1; 84 3.15,3.1; 85 5.25,3.1; 86 7.35,3.1; 87 1.05,5.15; 88 3.15,5.15; 89 5.25,5.15; 90 7.35,5.15; 91 1.05,-5.15; 92 3.15,-5.15; 93 5.25,-5.15; 94 7.35,-5.15; 95 1.05,-3.1; 96 3.15,-3.1; 97 5.25,-3.1; 98 7.35,-3.1; 99 1.05,-1.05; 100 3.15,-1.05; 101 5.25,-1.05; 102 7.35,-1.05
PAD.03X.05 = smd 1.27 x 1.27: 1 0,0

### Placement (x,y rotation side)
!SAFEBOOT_NEO!  12.7,34.29 0 top
!SAFEBOOT_ZED!  35.56,20.32 0 top
BT1  32.89,46.29 180 top
C1  33.08,36.2 0 top
C2  39.37,47.62 180 top
C3  14.86,52.77 90 top
C4  39.37,41.27 0 top
C5  39.37,39.37 180 top
C6  20.76,33.66 270 top
C7  29.65,31.75 180 top
C8  26.04,8.26 90 top
C9  20.89,8.26 270 top
C10  22.48,8.26 90 top
C11  22.29,33.66 90 top
D1  33.91,31.18 270 top
D2  3.17,8.89 270 top
D3  34.92,41.91 0 top
D4  3.17,54.61 90 top
D5  38.1,50.8 90 top
D6  40.64,50.8 90 top
FB1  32.26,32.58 90 top
FRAME2  not placed on the board
GEO  8,34.29 0 bottom
I2C  12.7,53.34 0 bottom
J1  39.37,31.75 270 top
J2  8.89,58.42 180 top
J3  6.35,16.51 270 top
J4  8.89,5.08 0 top
J5  1.27,24.13 90 top
J6  6.35,46.99 270 top
J7  24.13,62.23 0 top
J8  24.13,1.27 0 top
J9  21.59,62.23 180 top
J10  13.97,1.27 0 top
JP21  42.55,0.64 0 top
JP31  2.54,60.93 0 top
JP41  40.64,60.93 0 top
JP61  0.64,62.84 0 top
JP71  42.55,0.64 0 bottom
JP81  0.64,62.84 0 bottom
JP91  2.54,2.54 0 top
JP101  40.64,2.54 0 top
L1  35.56,32.64 90 top
LED1  8.38,26.67 180 top
LED2  8.38,31.75 180 top
LED3  8.38,34.29 180 top
LED4  8.38,36.83 180 top
LOGO1  OSHW-LOGOS  [OSHW-LOGO-S]  30.48,53.34 270 top
LOGO4  12.95,21.59 90 bottom
LOGO5  not placed on the board
PWR\  8,26.67 0 bottom
R1  8.38,24.13 0 top
R2  20.95,52.77 90 top
R3  17.91,52.77 90 top
R4  19.43,52.77 90 top
R5  16.19,33.66 270 top
R6  16.38,52.77 90 top
R7  11.81,52.77 270 top
R8  13.34,52.77 270 top
R9  19.24,33.66 90 top
R10  17.72,33.66 90 top
R11  14.67,33.66 270 top
R12  9.53,15.37 180 top
R13  9.53,18.29 180 top
R14  31.37,38.73 180 top
R15  29.21,8.26 90 top
R16  27.62,8.26 90 top
R17  9.53,12.19 180 top
R18  9.53,13.78 180 top
R19  36.2,14.61 0 top
R20  36.2,16.19 0 top
R21  36.2,11.43 0 top
R22  36.2,13.02 0 top
R23  9.53,19.88 180 top
R24  9.53,21.46 180 top
R25  36.2,24.57 0 top
R26  36.2,17.78 0 top
R27  8.38,29.21 180 top
R28  9.53,42.93 0 top
R29  9.53,41.27 180 top
R30  36.2,22.99 0 top
R31  22.48,52.77 90 top
R32  31.11,41.91 0 top
R33  9.53,44.58 180 top
R34  9.53,46.23 180 top
RTK  8,31.75 0 bottom
RX2-TX2  24.13,55.24 0 bottom
SHLD_NEO  1.78,46.99 0 bottom
SHLD_ZED  1.78,16.51 0 bottom
TP  8,36.83 0 bottom
TX2-RX2  26.67,55.24 0 bottom
U1  20.32,43.18 270 top
U2  39.37,44.45 180 top
U3  26.67,31.75 270 top
U4  22.86,19.05 180 top
U$1  [#GND#0]  21.59,61.47 270 top
U$2  [#GND#0]  2.03,24.13 0 top
U$3  [#GND#0]  13.97,2.03 90 bottom
U$4  [#GND#1]  13.97,2.03 270 top
U$5  [#GND#1]  2.03,24.13 0 bottom
U$6  [#GND#1]  21.59,61.47 90 bottom
U$7  [#SHLD#0]  3.68,46.99 90 bottom
U$8  [#SDA#0]  16.51,61.47 270 top
U$9  [#SCL#0]  21.59,2.03 90 bottom
U$10  [#SDA#0]  19.05,2.03 90 bottom
U$11  [#SDA#1]  19.05,2.03 270 top
U$12  [#SDA#1]  16.51,61.47 90 bottom
U$13  [#SCL#0]  13.97,61.47 270 top
U$14  [QWIIC_4MM]  8.89,6.63 0 top
U$15  [#SCL#1]  13.97,61.47 90 bottom
U$16  [#RTK#0]  2.03,31.75 0 top
U$17  [#RTK#1]  2.03,31.75 0 bottom
U$18  [#GEO#0]  2.03,34.29 0 top
U$19  [#GEO#1]  2.03,34.29 0 bottom
U$20  [#5V#0]  2.03,29.21 0 top
U$21  [#5V#6]  2.03,29.21 0 bottom
U$22  [#3V3#0]  19.05,61.47 270 top
U$23  [#3V3#0]  16.51,2.03 90 bottom
U$24  [#3V3#4]  19.05,61.47 90 bottom
U$25  [#3V3#4]  16.51,2.03 270 top
U$26  [#TP#0]  2.03,36.83 0 top
U$27  [#TP#1]  2.03,36.83 0 bottom
U$28  [#TX_RDY#0]  2.03,39.37 0 top
U$29  [#TX_RDY#1]  2.03,39.37 0 bottom
U$30  [#SCL#1]  21.59,2.03 270 top
U$31  [#TX2#0]  26.67,54.61 90 bottom
U$32  [#RX2#0]  24.13,54.61 90 bottom
U$33  [OPEN_JUMPERS_TO0]  26.42,43.81 90 bottom
U$34  [#RX2#0]  24.13,2.03 270 top
U$35  [#RX2#0]  26.67,61.47 90 bottom
U$36  [#RX2#3]  26.67,61.47 270 top
U$37  [#RX2#3]  24.13,2.03 90 bottom
U$38  [QWIIC_4MM]  8.89,56.79 0 top
U$39  [#TX2#0]  26.67,2.03 270 top
U$40  [#TX2#0]  24.13,61.47 90 bottom
U$41  [#TX2#3]  24.13,61.47 270 top
U$42  [#TX2#3]  26.67,2.03 90 bottom
U$43  [#RX1#0]  29.21,2.03 270 top
U$44  [#RX1#0]  31.75,61.47 90 bottom
U$45  [##RESET##0]  36.83,2.03 270 top
U$46  [##RESET##1]  36.83,2.03 90 bottom
U$47  [#EXT_INT#0]  34.29,2.03 270 top
U$48  [#EXT_INT_ZED#0]  34.29,2.03 90 bottom
U$49  [#RX1#2]  31.75,61.47 270 top
U$50  [#RX1#2]  29.21,2.03 90 bottom
U$51  [#TX1#0]  31.75,2.03 270 top
U$52  [#I�C#0]  10.48,53.34 90 bottom
U$53  [#SHLD#0]  3.68,16.51 90 bottom
U$54  [ISOLATE_UART21]  24.38,44.45 90 bottom
U$55  [NEO#D9S0]  21.59,21.59 90 bottom
U$56  [#3V3#0]  2.03,26.67 0 top
U$57  [#TX1#0]  29.21,61.47 90 bottom
U$58  [#ANT_PWR#0]  36.83,61.47 90 bottom
U$59  [#ANT_PWR#1]  36.83,61.47 270 top
U$60  [#TX1#2]  29.21,61.47 270 top
U$61  [#TX1#2]  31.75,2.03 90 bottom
U$62  [#EXT_INT_NEO#0]  34.29,61.47 270 top
U$63  [#EXT_INT_NEO#1]  34.29,61.47 90 bottom
U$64  [ZED#F9P0]  24.13,21.59 90 bottom
U$65  [ZED#F9P10]  1.27,7.62 270 top
U$66  [NEO#D9S10]  1.27,55.63 270 top
U$67  [COMBO10]  19.05,21.59 90 bottom
U$68  [BREAKOUT11]  16.51,21.59 90 bottom
U$69  [#PWR#0]  8.89,26.67 0 bottom
U$70  [#3V3#4]  2.03,26.67 0 bottom
U$71  [#SAFEBOOT#_NEO0]  12.7,34.67 90 bottom
U$72  [#SAFEBOOT#_ZED0]  35.56,20.7 90 bottom
U$73  [NEO#D9S_DEF_ADDR#_0X4310]  16.51,46.99 90 bottom
U$74  [ZED#F9P_DEF_ADDR#_0X420]  17.91,47.12 90 bottom
U$75  [ZED#F9P_NEO#D9S_COMBO_BREAKOUT0]  23.75,29.21 0 top
U$76  [V_BKCP0]  34.54,45.72 90 bottom
U$77  40.64,19.05 270 top
U$78  27.3,21.59 90 bottom
V_BKCP  33.02,45.72 0 bottom

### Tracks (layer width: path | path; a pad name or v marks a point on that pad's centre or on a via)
3.3V  (via drill 0.3)
  Top 0.508: J9.2 v19.05,56.64 | 9.39,56.65 J2.2 v9.39,59.68 v9.4,59.69 | 9.39,56.65 v10.16,55.88 | J5.2 3.81,26.67 v5.08,25.4 | R1.2 v10.79,24.13 | v8.64,55.88 8.64,55.9 9.39,56.65 | v14.35,47.75 14.42,47.82 U1.23 14.42,50.74 14.86,51.18 C3.1 | U1.22 15.52,47.85 v15.62,47.75 | C4.1 37.88,41.91 v37.21,41.91 D3.A | C4.1 C5.2 v37.34,39.37 | C4.1 39.37,42.12 39.37,42.8 39.72,43.15 U2.5 41.24,43.15 v41.27,43.18 | 20.83,9.17 C9.1 20.89,9.84 v21.21,10.16 U4.33 | U4.38 26.71,10.2 v26.67,10.16 26.04,9.53 C8.2 | v19.88,38.67 19.92,38.63 U1.7 19.92,36.59 20.77,35.75 C6.1 C11.2 | v8.38,3.94 J4.2 | U4.34 22.31,10.2 v22.35,10.16 22.48,10.03 C10.2
  Bottom 0.508: I2C.2 v12.7,54.77
  pour Route15 (isolate 0.203): 0,0 0,63.5 43.18,63.5 43.18,0
5V  (via drill 0.3)
  Top 0.406: v41.91,50.8 v41.91,49.53 41.79,49.65 D6.C | D5.C D6.C | D6.C 40.64,48.05 C2.1 40.32,47.52 U2.1 40.32,44.38 40.07,44.13 38.8,44.13 38.42,44.51 U2.3
  Route15 0.406: J5.3 3.05,30.99 3.05,38.86 3.81,39.62 3.81,45.47 2.64,46.64 2.64,51.97 1.78,52.83 1.78,56.52 3.96,58.7 38.58,58.7 41.91,55.36 v41.91,50.8 v41.91,49.53
!RESET!  (via drill 0.3)
  Top 0.152: U1.8 22.92,35.59 v22.95,35.56 | v34.23,20.13 32.83,20.13 U4.49
  Bottom 0.152: v22.95,35.56 22.75,35.36 22.75,30.83 20.98,29.07 14.79,29.07 14.48,28.77 14.48,11.31 16.75,9.04 23.65,9.04 24.03,9.43 24.03,10.36 25.1,11.43 33.02,11.43 | 33.02,11.43 34.23,12.64 v34.23,20.13 | 33.02,11.43 36.83,7.62 J8.6
!SAFEBOOT_NEO!
  Top 0.152: U1.1 13.32,36.69 12.7,36.07 !SAFEBOOT_NEO!.1
!SAFEBOOT_ZED!
  Top 0.152: U4.50 34.63,21.25 !SAFEBOOT_ZED!.1
ANT
  Top 0.318: C7.2 27.94,31.75 U3.2
ANT_NEO
  Top 0.318: U3.4 26.19,37.15 U1.11
ANT_PWR  (via drill 0.3)
  Top 0.406: L1.2 v35.56,34.92
  Bottom 0.406: J7.6 36.83,54.61 35.56,53.34 35.56,37.27 36.01,36.83 36.01,35.37 v35.56,34.92
ANT_VCC
  Top 0.406: FB1.2 32.23,33.45 C1.1 R14.1
ANT_ZED
  Top 0.318: U4.2 28.91,28.24 arc90 27.94,29.21 26.92,29.21 arc-90 26.19,29.95 U3.6
D+_NEO  (via drill 0.3)
  Top 0.254: v2.57,55.82 2.67,55.71
  Top 0.267: R9.1 19.24,32.58 18.54,31.88 v18.54,31.62 | 2.67,55.71 D4.6
  Bottom 0.267: v18.54,31.62 18.41,31.75 18.41,41.4 8.13,51.69 8.13,53.59 6.6,55.12 5.46,55.12 4.16,56.42 3.37,56.42 2.76,55.82 v2.57,55.82
D+_ZED  (via drill 0.3)
  Top 0.254: 3.75,7.81 3.67,7.88
  Top 0.267: R15.1 v29.21,6.35 | v3.75,7.11 3.75,7.81 | 3.67,7.88 D2.6
  Bottom 0.267: v29.21,6.35 28.48,6.35 27.81,7.02 3.84,7.02 v3.75,7.11
D-_NEO  (via drill 0.3)
  Top 0.267: D4.4 3.67,55.71 v3.78,55.82 | R10.1 v17.72,31.62
  Bottom 0.267: v17.72,31.62 17.84,31.75 17.84,41.21 7.59,51.46 7.59,53.37 6.35,54.61 5.24,54.61 4.04,55.82 v3.78,55.82
D-_ZED  (via drill 0.3)
  Top 0.267: R16.1 v27.62,6.35 | v2.6,7.11 2.6,7.81 2.67,7.88 D2.4
  Bottom 0.267: v2.6,7.11 3.24,6.48 27.5,6.48 v27.62,6.35
EXT_INT_NEO
  Top 0.152: R31.2 32.03,53.62 34.29,55.88 J7.5
EXT_INT_ZED  (via drill 0.3)
  Top 0.152: R30.2 39.22,20.81 39.22,7.16 36.88,4.82 v35.56,4.82
  Bottom 0.152: v35.56,4.82 34.29,3.55 J8.5
GEO  (via drill 0.3)
  Top 0.152: R28.2 10.41,42.93 11.43,41.91 11.43,39.37 10.16,38.1 7.03,38.1 6.13,37.2 6.13,34.29 | 6.13,34.29 v6.13,33.02 | J5.5 6.13,34.29 | R24.2 7.51,21.46 6.67,22.3 6.67,25.08 v7.05,25.46
  Bottom 0.152: v7.05,25.46 6.16,26.35 6.16,32.99 v6.13,33.02
GND  (via drill 0.3)
  Top 0.254: D2.2 3.17,10.3 v3.22,10.35 | D4.2 3.17,53.51 v3.08,53.41
  Top 0.406: U2.2 v39.37,44.74
  Top 0.508: v10.41,59.69 10.41,58.44 J2.1 10.39,56.92 v11.43,55.88
  other vias: 25.4,31.75 27.94,33.02 27.94,30.48 25.4,30.48 25.4,33.02 25.08,34.29 25.08,35.43 27.3,35.43 27.3,34.29 25.4,29.21 27.81,28.07 26.16,28.07 29.97,28.19 30.48,30.48 32.26,30.48 30.48,33.02 33.91,29.59 35.31,36.2 40.64,27.94 38.1,27.94 36.83,29.21 35.37,29.59 40.64,35.56 38.1,35.56 36.83,34.29 25.15,38.67 27.43,38.67 30.48,36.13 34.29,38.1 33.02,40.64 30.48,40.64 27.94,40.64 25.4,40.64 23.5,34.29 23.37,40.64 23.5,31.75 23.24,28.57 31.24,26.67 16.38,23.18 20.76,23.18 24.96,23.18 29.15,23.18 29.21,19.05 24.89,19.05 20.76,19.05 15.24,19.05 29.15,14.92 24.96,14.92 20.7,14.92 16.51,14.67 31.62,19.05 19.88,10.16 25.46,10.16 30.04,10.16 15.68,27.94 17.91,27.94 30.48,34.61 33.97,34.92 33.97,33.27 35.43,26.8 8.06,27.94 8.06,30.48 8.06,33.02 8.06,35.56 11.62,46.23 11.62,44.58 13.4,47.75 14.8,54.86 27.37,47.75 36.83,48.26 36.83,46.99 41.53,41.27 41.53,39.37 31.75,49.53 7.43,3.81 6.35,5.08 19.88,7.62 24.89,7.62 2.54,17.78 2.54,15.24 2.54,45.72 6.99,43.75 7.05,50.23 6.99,19.81 6.99,13.27 11.43,15.37 11.43,18.29 20.76,31.69 1.27,5.08 15.24,59.69 25.4,59.69 29.21,55.88 31.75,55.88 15.24,45.72 20.32,45.72 22.86,45.72 27.94,45.72 27.94,43.18 22.86,43.18 20.32,43.18 13.97,43.18 13.97,39.37 15.24,39.37 20.32,40.64 40.64,21.59 36.83,19.05 40.64,16.51 40.64,12.7 40.64,8.89 35.56,10.16 33.02,3.81 25.4,3.81 8.89,1.27 13.97,8.89 6.35,8.89 5.08,57.15 5.08,53.34 8.89,62.23 29.21,50.8 8.89,39.37 17.78,19.05 23.62,7.62
  pour Top (isolate 0.203): 0,63.5 43.18,63.5 43.18,0 0,0
  pour Bottom (isolate 0.203): 0,63.5 43.18,63.5 43.18,0 0,0
  pour Top (isolate 0.127): 22.86,40.64 22.86,24.13 43.18,24.13 43.18,40.64
  pour Route2 (isolate 0.203): 0,63.5 43.18,63.5 43.18,0 0,0
N$1  (via drill 0.3)
  Top 0.152: v8,25.27 7.53,24.8 R1.1
  Bottom 0.152: v8,25.27 7.48,25.79 PWR\.2
N$2
  Top 0.152: U1.20 17.72,51.73 R3.1
N$3
  Top 0.152: R2.1 20.95,50.67 19.92,49.64 U1.18
N$4
  Top 0.152: R4.1 19.43,51.05 18.82,50.44 U1.19
N$5  (via drill 0.3)
  Top 0.152: R8.2 13.34,51.18 12.95,50.8 v12.7,50.8
  Bottom 0.152: v12.7,50.8 13.51,51.61 I2C.1
N$6
  Top 0.152: U1.21 16.62,51.68 R6.1
N$7
  Top 0.152: J3.B5 7.14,14.76 7.75,15.37 R12.2
N$8  (via drill 0.3)
  Top 0.152: R7.2 10.69,50.8 v10.67,50.8
  Bottom 0.152: v10.67,50.8 11.89,52.02 I2C.3
N$9
  Top 0.152: J3.A5 7.03,17.76 7.56,18.29 R13.2
N$10  (via drill 0.3)
  Top 0.152: LED1.A 9.26,25.91 9.77,25.4 v10.16,25.4
  Bottom 0.152: v10.16,25.4 10.16,26.18 9.66,26.67 PWR\.1
N$11
  Top 0.267: U1.6 18.82,35.79 19.24,35.37 R9.2
N$12
  Top 0.267: U1.5 R10.2
  Top 0.406: R10.2
N$13
  Top 0.406: D3.C R32.2
N$14
  Top 0.152: R11.1 14.67,35.31 15.52,36.16 U1.3
N$15
  Top 0.152: R5.1 16.19,35.31 16.62,35.73 U1.4
N$16
  Top 0.267: U4.40 28.91,9.4 R15.2
N$17
  Top 0.267: U4.39 27.81,9.29 R16.2
N$18
  Top 0.152: U4.44 35.3,14.65 R19.1
N$19
  Top 0.152: U4.45 33.97,15.75 34.42,16.19 R20.1
N$20
  Top 0.152: U4.42 32.81,11.77 33.15,11.43 R21.1
N$21
  Top 0.152: U4.43 34.81,13.55 R22.1
N$22
  Top 0.152: U4.46 34.31,16.85 35.24,17.78 R26.1
N$23  (via drill 0.3)
  Top 0.152: v10.79,31.75 LED2.A
  Bottom 0.152: RTK.1 v10.79,31.75
N$24
  Top 0.152: U4.27 11.62,12.45 11.37,12.19 R17.1
N$25
  Top 0.152: U4.26 11.66,13.55 11.43,13.78 R18.1
N$26  (via drill 0.3)
  Top 0.152: v10.79,34.29 LED3.A
  Bottom 0.152: GEO.1 v10.79,34.29
N$27  (via drill 0.3)
  Top 0.152: v10.73,36.83 LED4.A
  Bottom 0.152: TP.1 v10.73,36.83
N$28  (via drill 0.3)
  Top 0.152: R27.1 v10.79,29.21
  Bottom 0.152: RTK.2 7.48,29.73 8,29.21 v10.79,29.21
N$29  (via drill 0.3)
  Top 0.152: R28.1 v7.56,42.93
  Bottom 0.152: v7.56,42.93 7.56,41.85 5.93,40.22 5.93,34.71 6.35,34.29 GEO.2
N$30  (via drill 0.3)
  Top 0.152: R29.1 10.16,41.06 v10.16,39.37
  Bottom 0.152: v10.16,39.37 9.27,38.48 7.87,38.48 7.48,38.09 TP.2
N$31
  Top 0.152: U4.51 33.91,22.35 34.54,22.99 R30.1
N$32
  Top 0.152: R31.1 22.48,51.18 22.92,50.74 U1.17
N$33
  Top 0.152: J6.B5 6.77,45.24 7.43,44.58 R33.2
N$34
  Top 0.152: J6.A5 7,48.24 7.62,47.62 7.62,46.42 7.81,46.23 R34.2
N$35
  Top 0.152: U4.20 11.64,20.15 11.37,19.88 R23.1
N$36
  Top 0.152: U4.19 11.77,21.25 11.56,21.46 R24.1
N$37
  Top 0.152: U4.53 35.32,24.55 R25.1
RTK
  Top 0.152: J5.4 5.5,31.75 6.31,30.94 6.31,29.21 | R23.2 8.68,19.9 6.31,22.26 6.31,29.21 | R27.2 6.31,29.21
RXD1_NEO  (via drill 0.3)
  Top 0.152: R6.2 16.38,54.48 17.93,56.03 26.82,56.03 27.94,57.15 v27.94,59.69
  Bottom 0.152: v27.94,59.69 30.48,59.69 31.75,60.96 J7.4
RXD1_ZED  (via drill 0.3)
  Top 0.152: R22.2 38.1,11.96 38.1,7.62 36.73,6.25 30.58,6.25 v30.48,6.35
  Bottom 0.152: v30.48,6.35 30.48,5.08 29.21,3.81 J8.3
RXD2_NEO  (via drill 0.3)
  Top 0.152: R5.2 15.75,32.36 v15.75,30.86
  Bottom 0.152: v15.75,30.86 16.7,29.91 20.64,29.91 21.91,31.18 21.91,47.82 26.15,52.06 TX2-RX2.2 26.15,59.17 26.67,59.69 J7.2
RXD2_ZED  (via drill 0.3)
  Top 0.152: R18.2 7.62,12.72 v7.62,10.03 7.62,9.84 13.69,3.77 19.6,3.77 20.83,2.54 22.86,2.54 J8.1
  Bottom 0.152: v7.62,10.03 12.43,10.03 13.64,11.24 13.64,29.44 15.55,31.34 16.12,31.34 17.24,30.23 20.51,30.23 21.59,31.3 21.59,47.99 24.65,51.05 RX2-TX2.1
SCL  (via drill 0.3)
  Top 0.152: J9.4 13.97,60.96 13.46,60.45 8.13,60.45 v7.37,59.69 7.39,59.67 J2.4 7.39,55.48 7.9,54.97 11.33,54.97 11.81,54.48 R7.1 | R4.2 v19.43,54.74 | J10.4 19.37,3.49 10.89,3.49 v10.41,3.97 10.41,5.06 J4.4 | R20.2 37.15,16.19 38.66,14.68 38.66,7.39 36.85,5.58 34.35,5.58 33.91,5.14 v22.86,5.14
  Bottom 0.152: v19.43,54.74 16.38,54.74 13.97,57.15 J9.4 | v7.37,59.69 6.38,58.7 2.81,58.7 0.99,56.88 0.99,54.3 3.53,51.76 3.53,12.37 0.99,9.83 0.99,6.23 2.11,5.12 4.65,5.12 6.93,2.83 9.27,2.83 v10.41,3.97 | v22.86,5.14 21.59,3.87 J10.4
SDA  (via drill 0.3)
  Top 0.152: J9.3 14.45,60.17 8.86,60.17 v8.38,59.69 v8.39,59.68 J2.3 8.39,56.65 7.87,56.13 7.87,55.5 8.13,55.24 13.08,55.24 13.34,54.99 R8.1 | v20.45,55.27 20.45,54.13 R2.2 | J10.3 19.05,2.79 18.73,3.11 10.22,3.11 v9.4,3.94 v9.39,3.94 J4.3 | R19.2 37.15,14.61 38.38,13.37 38.38,7.5 36.74,5.87 34.03,5.87 33.85,5.69 22.54,5.69 22.04,5.18 v20.38,5.18
  Bottom 0.152: v20.45,55.27 17.12,55.27 16.51,55.88 J9.3 | v9.4,3.94 8.57,3.11 7.05,3.11 4.76,5.4 2.22,5.4 1.27,6.35 1.27,9.72 3.81,12.26 3.81,51.94 1.27,54.48 1.27,56.64 3.05,58.42 7.11,58.42 v8.38,59.69 | v20.38,5.18 19.05,3.84 J10.3
SHIELD_NEO
  Route2 0.406: J6.SHLD3 J6.SHLD1 | J6.SHLD4 J6.SHLD2
  Bottom 0.406: J6.SHLD4 SHLD_NEO.2 J6.SHLD3
SHIELD_ZED
  Route2 0.406: J3.SHLD4 J3.SHLD2 | J3.SHLD3 J3.SHLD1
  Bottom 0.406: J3.SHLD3 SHLD_ZED.2 J3.SHLD4
SMA
  Top 0.318: J1.SIG 35.6,31.75 | 35.53,31.76 D1.1 | 33.88,31.73 FB1.1 30.53,31.73
  Top 0.813: 35.6,31.75 L1.1 35.53,31.76 | D1.1 33.88,31.73 | 30.53,31.73 C7.1
TP  (via drill 0.3)
  Top 0.152: J5.6 v5.08,36.83 5.08,38.61 7.75,41.27 R29.2 | R25.2 39.5,22.12 39.5,7.04 36.8,4.34 14.14,4.34 9.4,9.08 v9.4,10.79
  Bottom 0.152: v9.4,10.79 9.88,11.28 9.88,21.47 5.05,26.3 5.05,36.8 v5.08,36.83
TX_RDY  (via drill 0.3)
  Top 0.152: R26.2 38.94,15.89 38.94,7.27 36.97,5.3 34.51,5.3 33.87,4.66 14.27,4.66 9.78,9.14 9.78,10.41 v10.16,10.79 | v5.08,40.64 3.81,39.37 J5.7
  Bottom 0.152: v10.16,10.79 10.16,21.65 5.65,26.16 5.65,40.07 v5.08,40.64
TXD1_NEO
  Top 0.152: R3.2 17.91,54.99 18.67,55.75 27.05,55.75 29.21,57.91 J7.3
TXD1_ZED  (via drill 0.3)
  Top 0.152: R21.2 37.81,10.67 37.81,7.83 36.58,6.6 31.88,6.6 v31.75,6.73
  Bottom 0.152: v31.75,6.73 J8.4
TXD2_NEO  (via drill 0.3)
  Top 0.152: R11.2 v14.67,31.62
  Bottom 0.152: v14.67,31.62 14.7,31.66 16.2,31.66 17.35,30.5 20.39,30.5 21.31,31.42 21.31,48.23 23.61,50.53 RX2-TX2.2 23.61,59.17 24.13,59.69 J7.1
TXD2_ZED  (via drill 0.3)
  Top 0.152: R17.2 v8.68,9.53 8.68,9.3 13.92,4.05 19.76,4.05 20.89,2.92 25.02,2.92 J8.2
  Bottom 0.152: v8.68,9.53 8.8,9.65 12.45,9.65 13.92,11.13 13.92,29.19 14.36,29.63 20.75,29.63 22.19,31.06 22.19,47.59 27.19,52.59 TX2-RX2.1
USB_D+
  Top 0.254: 3.81,10.16 3.81,10.1
  Top 0.267: 3.81,10.16 3.81,15.24 4.33,15.76 J3.B6 6.74,15.76 6.99,16 6.99,16.51 6.74,16.76 J3.A6 | D2.1 3.67,9.96 3.81,10.1
USB_D+1
  Top 0.254: 2.67,53.82 2.48,53.63
  Top 0.267: J6.A6 5.08,47.24 | 5.08,47.24 4.07,47.24 3.11,48.2 3.11,52.58 2.48,53.2 2.48,53.63 | 2.67,53.82 D4.1 | J6.B6 5.32,46.24 5.08,46.48 5.08,47.24
USB_D-
  Top 0.254: D2.3 2.67,10.15 2.67,10.16
  Top 0.267: J3.A7 4.89,16.26 4.89,17.02 5.13,17.26 J3.B7 | 2.67,10.16 2.67,10.73 3.3,11.37 3.3,15.43 4.13,16.26
  Top 0.305: 4.89,16.26 4.13,16.26
USB_D-1
  Top 0.254: 3.67,52.59 3.68,52.58
  Top 0.267: D4.3 3.67,52.59 | 3.68,52.58 3.68,48.32 4.27,47.74 J6.B7 6.68,47.74 6.92,47.5 6.92,46.93 6.74,46.74 J6.A7
V_BKCP  (via drill 0.3)
  Top 0.152: R32.1 v29.21,41.91 | v24.51,10.16 U4.36
  Top 0.406: R32.1 30.27,43.65 BT1.+
  Bottom 0.152: v24.51,10.16 24.51,9.27 24,8.76 16.64,8.76 14.2,11.2 14.2,28.95 14.6,29.35 20.87,29.35 22.47,30.95 22.47,41.26 23.11,41.91 v29.21,41.91 29.21,44.45 30.48,45.72 V_BKCP.1
V_USB  (via drill 0.3)
  Top 0.254: D2.5 v3.17,7.62
  Top 0.406: D5.A v38.1,53.34 v38.1,54.61 | J3.VBUS2 5.5,14.06 v4.83,14.73 | J3.VBUS1 5.5,18.96 v4.83,18.29
  Route15 0.406: v38.1,53.34 v38.1,54.61 38.1,55.88 36.6,57.38 10.39,57.38 9.4,56.39 9.4,42.42 4.34,37.36 4.34,23.39 3.81,22.86 3.81,18.29 | v4.83,14.73 3.81,14.73 | 3.81,14.73 3.81,18.29 | v4.83,18.29 3.81,18.29 | 3.81,14.73 3.17,14.1 3.17,11.75 3.83,11.09 3.83,8.28 v3.17,7.62
V_USB_2  (via drill 0.3)
  Top 0.254: v3.17,57.02 D4.5
  Top 0.406: D6.A v40.64,53.34 v40.64,54.61 | J6.VBUS2 5.5,44.54 v4.95,45.09 | J6.VBUS1 5.5,49.44 v4.95,48.9
  Route15 0.406: v40.64,53.34 v40.64,54.61 40.64,55.88 38.48,58.04 4.19,58.04 v3.17,57.02 3.17,55.24 2.31,54.38 2.31,53.05 3.17,52.19 3.17,48.9 | v4.95,45.09 3.17,46.86 3.17,48.9 | v4.95,48.9 3.17,48.9
VCC_RF
  Top 0.406: R14.2 29.88,39.37 24.77,39.37 24,38.61 24,37.2 U1.9

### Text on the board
Bottom: x01
Milling: Route Out
Measures: Measurements in inches
tDocu: 1.6mm Thickness / 4-Layers / 1oz copper / Lead-Free HASL finish / Black soldermask / White silkscreen | Paul Clark

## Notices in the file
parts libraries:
SparkFun-Resistors: Licensing: Creative Commons ShareAlike 4.0 International - https://creativecommons.org/licenses/by-sa/4.0
SparkFun-Aesthetics: Released under the Creative Commons Attribution Share-Alike 4.0 License
SparkFun-Aesthetics: https://creativecommons.org/licenses/by-sa/4.0
